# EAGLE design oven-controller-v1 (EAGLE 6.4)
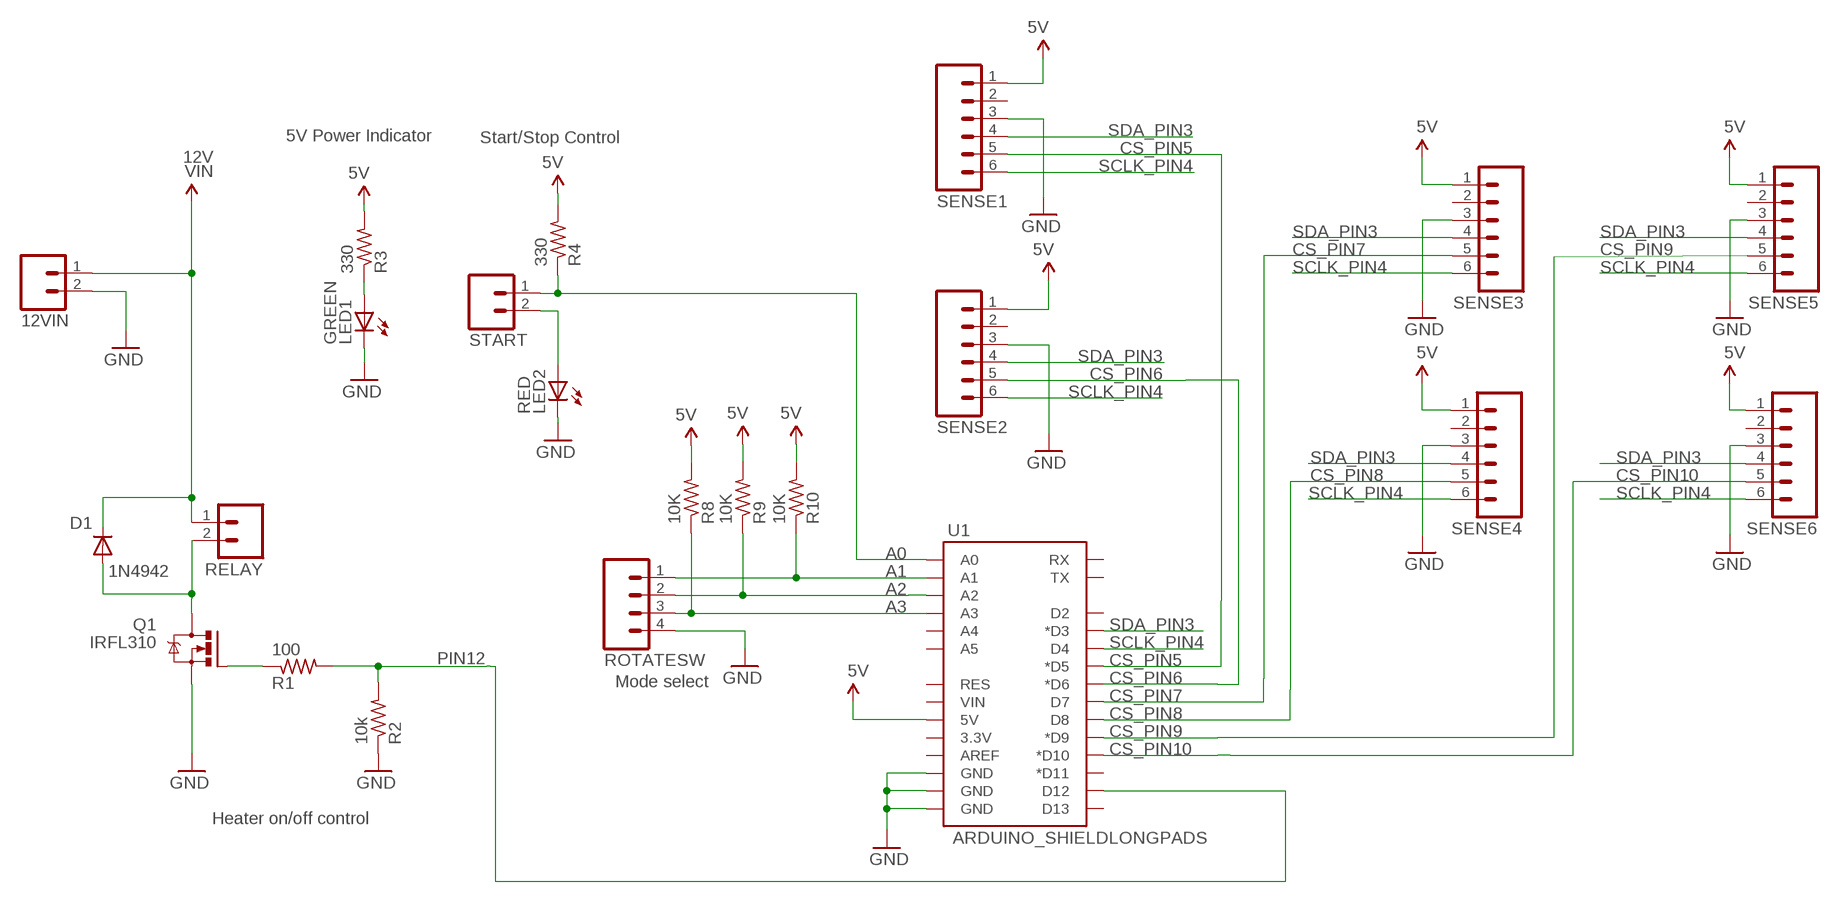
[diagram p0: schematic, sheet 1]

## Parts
12VIN  M023.5MM_LOCK  [SCREWTERMINAL-3.5MM-2_LOCK]
D1  1N4942  [DO41-10]
LED1  GREEN  LED5MM  [LED5MM]
LED2  RED  LED5MM  [LED5MM]
Q1  IRFL310  IRF520  [TO220BV]
R1  100  R-US_V234/12  [V234/12]
R2  10k  R-US_V234/12  [V234/12]
R3  330  R-US_0207/10  [0207/10]
R4  330  R-US_0207/10  [0207/10]
R8  10K  R-US_0207/10  [0207/10]
R9  10K  R-US_0207/10  [0207/10]
R10  10K  R-US_0207/10  [0207/10]
RELAY  M023.5MM_LOCK  [SCREWTERMINAL-3.5MM-2_LOCK]
ROTATESW  M04LOCK_LONGPADS  [1X04_LOCK_LONGPADS]
SENSE1  M06LOCK_LONGPADS  [1X06_LOCK_LONGPADS]
SENSE2  M06LOCK_LONGPADS  [1X06_LOCK_LONGPADS]
SENSE3  M06LOCK_LONGPADS  [1X06_LOCK_LONGPADS]
SENSE4  M06LOCK_LONGPADS  [1X06_LOCK_LONGPADS]
SENSE5  M06LOCK_LONGPADS  [1X06_LOCK_LONGPADS]
SENSE6  M06LOCK_LONGPADS  [1X06_LOCK_LONGPADS]
START  M023.5MM_LOCK  [SCREWTERMINAL-3.5MM-2_LOCK]
U1  ARDUINO_SHIELDLONGPADS  [DUEMILANOVE_SHIELD_LONGPADS]

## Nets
5V: R3.2 R4.2 R8.2 R9.2 R10.2 SENSE1.1 SENSE2.1 SENSE3.1 SENSE4.1 SENSE5.1 SENSE6.1 U1.5V
A0: R4.1 START.1 U1.A0
A1: R10.1 ROTATESW.1 U1.A1
A2: R9.1 ROTATESW.2 U1.A2
A3: R8.1 ROTATESW.3 U1.A3
CS_PIN5: SENSE1.5 U1.D5(*D5)
CS_PIN6: SENSE2.5 U1.D6(*D6)
CS_PIN7: SENSE3.5 U1.D7
CS_PIN8: SENSE4.5 U1.D8
CS_PIN9: SENSE5.5 U1.D9(*D9)
CS_PIN10: SENSE6.5 U1.D10(*D10)
GND: 12VIN.2 LED1.K(C) LED2.K(C) Q1.S R2.1 ROTATESW.4 SENSE1.3 SENSE2.3 SENSE3.3 SENSE4.3 SENSE5.3 SENSE6.3 U1.GND@0(GND) U1.GND@1(GND) U1.GND@2(GND)
N$2: Q1.G R1.1
N$3: D1.A Q1.D RELAY.2
N$10: LED2.A START.2
N$11: LED1.A R3.1
PIN12: R1.2 R2.2 U1.D12
SCLK_PIN4: SENSE1.6 SENSE2.6 SENSE3.6 SENSE4.6 SENSE5.6 SENSE6.6 U1.D4
SDA_PIN3: SENSE1.4 SENSE2.4 SENSE3.4 SENSE4.4 SENSE5.4 SENSE6.4 U1.D3(*D3)
VIN: 12VIN.1 D1.C RELAY.1
Unconnected: SENSE1.2 SENSE2.2 SENSE3.2 SENSE4.2 SENSE5.2 SENSE6.2 U1.3.3V U1.A4 U1.A5 U1.AREF U1.D2 U1.D11(*D11) U1.D13 U1.RES U1.RX U1.TX U1.VIN

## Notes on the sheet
- 5V Power Indicator | Start/Stop Control
- 12V
- Mode select
- Heater on/off control

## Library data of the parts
12VIN RELAY START = SparkFun-Connectors:M02: Header 2
D1 = diode:1N4942: DIODE
LED1 LED2 = led:LED: LED
Q1 = transistor-power:IRF520: HEXFET Power MOSFET
R1-R4 R8-R10 = resistor:R-US_: RESISTOR, American symbol
ROTATESW = SparkFun-Connectors:M04: Header 4 Standard 4-pin 0.1" header. Use with straight break away headers (SKU : PRT-00116), right angle break away headers (PRT-00553), swiss pins (PRT-00743), machine pins (PRT-00117), and female headers (PRT-00115). Molex polarized connector foot print use with SKU : PRT-08231 with associated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
SENSE1-SENSE6 = SparkFun-Connectors:M06: Header 6 Standard 6-pin 0.1" header. Use with straight break away headers (SKU : PRT-00116), right angle break away headers (PRT-00553), swiss pins (PRT-00743), machine pins (PRT-00117), and female headers (PRT-00115). Molex polarized connector foot print use with SKU : PRT-08094 with associated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
U1 = SparkFun-Boards:ARDUINO_SHIELD: Arduino shield footprint

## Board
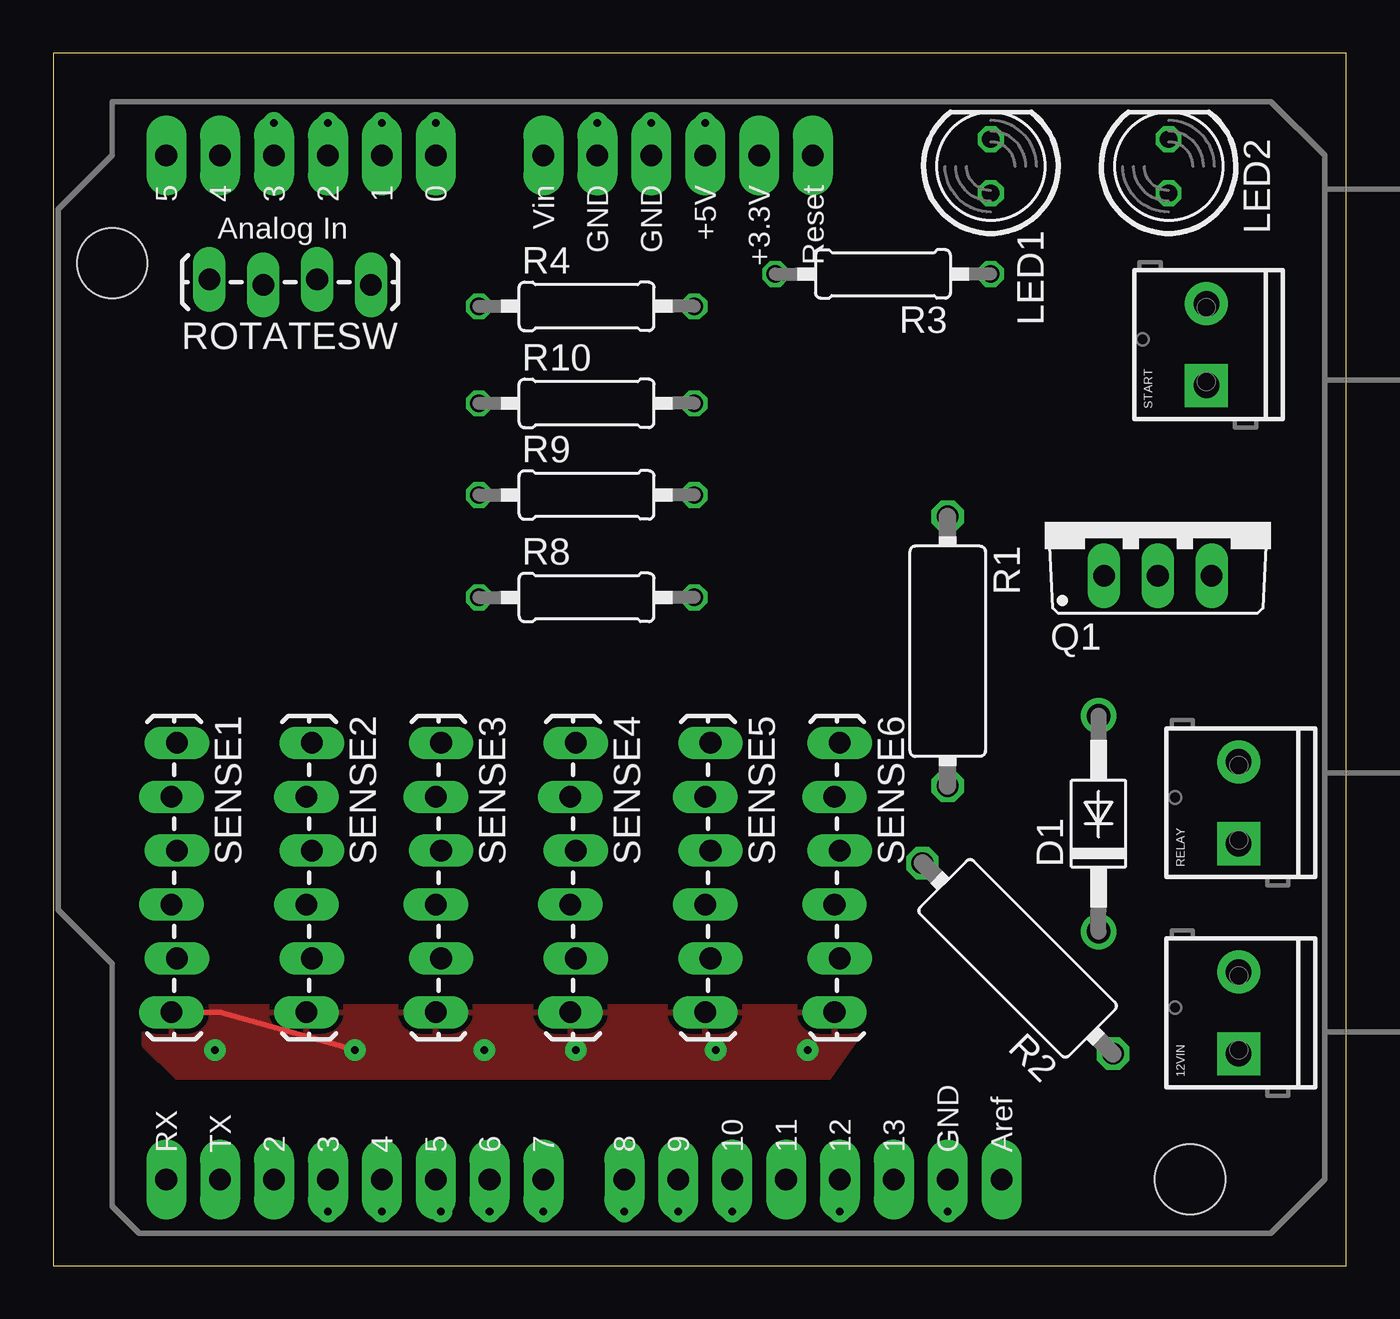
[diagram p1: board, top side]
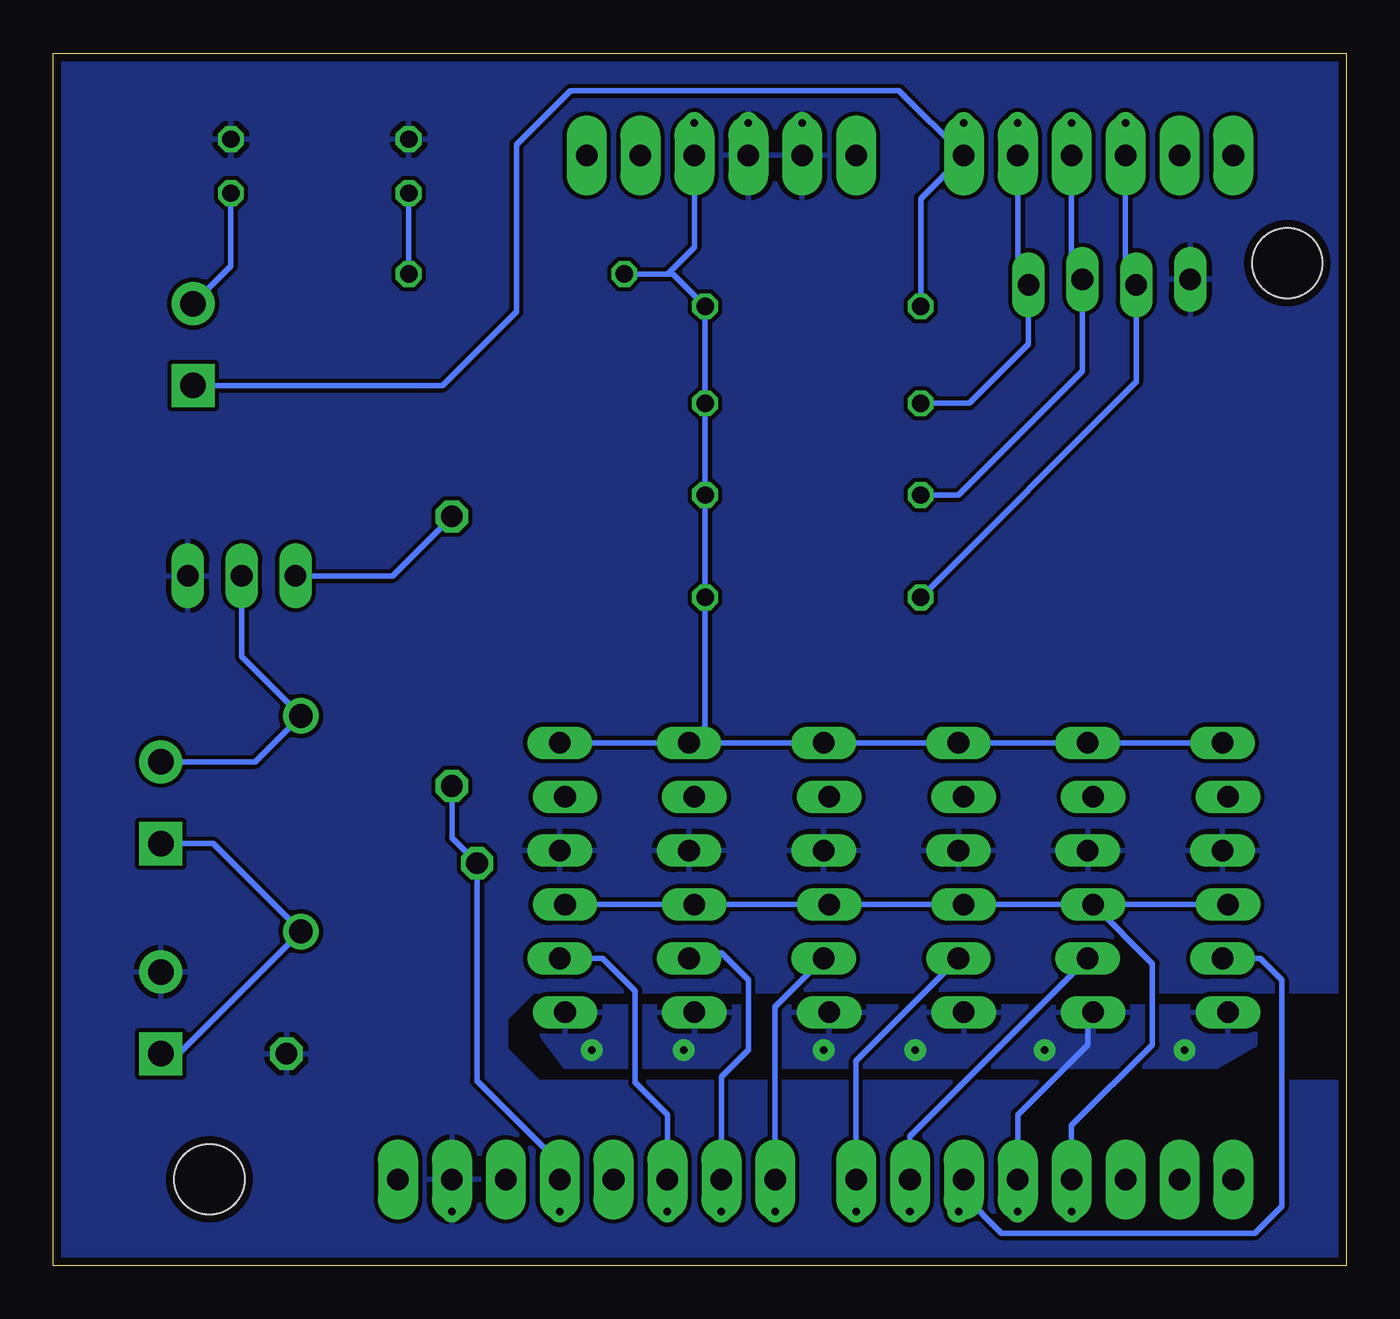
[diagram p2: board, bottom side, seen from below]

Size 60.96 x 57.15 mm. Coordinates in mm from the lower left corner, seen from the top.
Outline: 0,0 60.96,0 60.96,57.15 0,57.15 0,0
Copper layers (1*16): Top 0.0178mm / dielectric 59mil / Bottom 0.0178mm
Design rules "epl-lpkf": minimum track width 8mil, minimum drill 0.35mm, track to track 8mil, track to pad 8mil, pad to pad 8mil, via to via 8mil, smd to smd 8mil, copper to edge 15mil, drill to drill 15mil, minimum pad ring 8mil, minimum via ring 8mil, stop-mask expansion 3mil, vias tented up to drill 0mil, thermal gap 10mil

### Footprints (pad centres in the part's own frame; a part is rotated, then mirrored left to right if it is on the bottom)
SCREWTERMINAL-3.5MM-2_LOCK = drill 1.2 pad 2.032 square: 1 -0.178,0 | drill 1.2 pad 2.032: 2 3.678,0
DO41-10 = drill 1.118: A 5.08,0; C -5.08,0
LED5MM = drill 0.813 octagon: A -1.27,0; K 1.27,0
TO220BV = drill 1.016 long: D 0,-2.54; G -2.54,-2.54; S 2.54,-2.54
V234/12 = drill 1.016 octagon: 1 -6.35,0; 2 6.35,0
0207/10 = drill 0.813 octagon: 1 -5.08,0; 2 5.08,0
1X04_LOCK_LONGPADS = drill 1.016 long: 1 0,0; 2 2.54,-0.254; 3 5.08,0; 4 7.62,-0.254
1X06_LOCK_LONGPADS = drill 1.016 long: 1 0,0; 2 2.54,-0.254; 3 5.08,0; 4 7.62,-0.254; 5 10.16,0; 6 12.7,-0.254
DUEMILANOVE_SHIELD_LONGPADS = drill 1.016 pad 1.88 long: 3.3V 50.8,26.67; 5V 50.8,29.21; A0 50.8,41.91; A1 50.8,44.45; A2 50.8,46.99; A3 50.8,49.53; A4 50.8,52.07; A5 50.8,54.61; AREF 2.54,15.24; D2 2.54,49.53; D3 2.54,46.99; D4 2.54,44.45; D5 2.54,41.91; D6 2.54,39.37; D7 2.54,36.83; D8 2.54,33.02; D9 2.54,30.48; D10 2.54,27.94; D11 2.54,25.4; D12 2.54,22.86; D13 2.54,20.32; GND@0 50.8,31.75; GND@1 50.8,34.29; GND@2 2.54,17.78; RES 50.8,24.13; RX 2.54,54.61; TX 2.54,52.07; VIN 50.8,36.83 | hole 3.302: 45.72,57.15; 2.54,6.35

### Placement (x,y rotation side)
12VIN  55.88,10.16 90 top
D1  49.28,20.83 90 top
LED1  44.2,51.82 90 top
LED2  52.58,51.82 90 top
Q1  52.07,35.05 0 top
R1  42.16,28.96 270 top
R2  45.47,14.48 135 top
R3  39.12,46.74 180 top
R4  25.15,45.21 0 top
R8  25.15,31.5 0 top
R9  25.15,36.32 0 top
R10  25.15,40.64 0 top
RELAY  55.88,20.07 90 top
ROTATESW  14.99,46.23 180 top
SENSE1  5.84,24.64 270 top
SENSE2  12.19,24.64 270 top
SENSE3  18.29,24.64 270 top
SENSE4  24.64,24.64 270 top
SENSE5  30.99,24.64 270 top
SENSE6  37.08,24.64 270 top
START  54.36,41.66 90 top
U1  59.94,1.52 90 top

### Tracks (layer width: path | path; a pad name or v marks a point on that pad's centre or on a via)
5V  (via drill 0.36 pad 1.02)
  Bottom 0.254: SENSE1.1 SENSE2.1 SENSE3.1 SENSE4.1 SENSE5.1 | SENSE5.1 SENSE6.1 | R3.2 32,46.74 | 32,46.74 31.75,46.74 R4.2 R10.2 R9.2 R8.2 30.23,25.4 SENSE5.1 | 32,46.74 30.73,48.01 U1.5V v30.73,53.85
A0  (via drill 0.36 pad 1.02)
  Bottom 0.254: START.1 42.6,41.48 39.12,44.96 39.12,52.83 36.58,55.37 21.08,55.37 U1.A0 | R4.1 20.07,50.29 U1.A0 | v18.03,53.85 U1.A0
A1  (via drill 0.36 pad 1.02)
  Bottom 0.254: R10.1 17.78,40.64 14.99,43.43 ROTATESW.1 15.49,46.74 U1.A1 v15.49,53.85
A2  (via drill 0.36 pad 1.02)
  Bottom 0.254: R9.1 18.29,36.32 12.45,42.16 ROTATESW.2 12.95,46.99 U1.A2 v12.95,53.85
A3  (via drill 0.36 pad 1.02)
  Bottom 0.254: R8.1 9.91,41.66 ROTATESW.3 10.41,46.74 U1.A3 v10.41,53.85
CS_PIN5  (via drill 0.36 pad 1.02)
  Bottom 0.254: U1.D5 18.03,3.3 | 18.03,3.3 16.26,1.52 4.32,1.52 4.06,1.78 | 4.06,1.78 3.56,2.29 | SENSE1.5 4.06,14.48 3.05,13.46 3.05,2.79 4.06,1.78 | v18.29,2.54 18.03,2.54 18.03,3.3
CS_PIN6  (via drill 0.36 pad 1.02)
  Bottom 0.254: SENSE2.5 20.57,6.1 U1.D6 v20.57,2.54
CS_PIN7  (via drill 0.36 pad 1.02)
  Bottom 0.254: SENSE3.5 23.11,9.65 U1.D7 v23.11,2.54
CS_PIN8  (via drill 0.36 pad 1.02)
  Bottom 0.254: SENSE4.5 26.92,12.19 U1.D8 v26.92,2.54
CS_PIN9  (via drill 0.36 pad 1.02)
  Bottom 0.254: SENSE5.5 30.73,14.73 29.46,14.73 28.19,13.46 28.19,10.16 29.46,8.89 U1.D9 v29.46,2.54
CS_PIN10  (via drill 0.36 pad 1.02)
  Bottom 0.254: SENSE6.5 35.05,14.48 33.53,12.95 33.53,8.64 32,7.11 U1.D10 v32,2.54
GND  (via drill 0.36 pad 1.02)
  other vias: 25.65,53.85 28.19,53.85 42.16,2.54
  pour Bottom: 61.21,57.66 -0.76,57.66 -1.02,13.72 -0.25,12.95 38.35,12.95 39.62,11.68 39.62,10.16 38.1,8.64 0.51,8.64 -1.02,7.11 -1.02,0 60.96,0
N$2
  Bottom 0.254: Q1.G 44.96,32.51 R1.1
N$3
  Bottom 0.254: RELAY.2 51.44,23.74 D1.A 52.07,28.7 Q1.D
N$10
  Bottom 0.254: LED2.A 52.58,47.11 START.2
N$11
  Bottom 0.254: LED1.A R3.1
PIN12  (via drill 0.36 pad 1.02)
  Bottom 0.254: R1.2 42.16,20.16 R2.2 40.98,8.72 40.01,7.75 | 40.01,7.75 37.08,4.83 U1.D12 v37.08,2.54 | 40.01,7.75 40.39,8.13
SCLK_PIN4  (via drill 0.36 pad 1.02)
  Top 0.254: SENSE5.6 30.99,11.94 | SENSE1.6 7.87,11.94 v14.22,10.16
  Bottom 0.254: SENSE2.6 12.19,11.68 12.19,10.41 15.49,7.11 U1.D4 v15.49,2.54
  other vias: 7.62,10.16 20.32,10.16 24.64,10.16 31.24,10.16 35.56,10.16
  pour Top: 4.32,11.94 4.32,10.41 5.84,8.89 36.58,8.89 38.35,11.43 37.59,12.19 4.57,12.19
  pour Bottom: 4.32,11.94 4.32,10.41 6.1,9.4 36.83,9.4 38.35,11.43 37.59,12.19 4.57,12.19
SDA_PIN3  (via drill 0.36 pad 1.02)
  Bottom 0.254: SENSE2.4 9.14,14.22 9.14,10.41 12.95,6.6 U1.D3 v12.95,2.54 | SENSE1.4 SENSE2.4 | SENSE2.4 SENSE3.4 SENSE4.4 SENSE5.4 SENSE6.4
VIN
  Bottom 0.254: RELAY.1 53.42,19.89 D1.C 55.04,9.98 12VIN.1

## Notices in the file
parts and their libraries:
SparkFun-Boards: Licensing: CC v3.0 Share-Alike You are welcome to use this library for commercial purposes.
